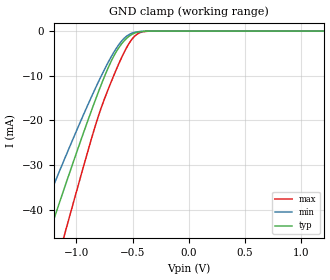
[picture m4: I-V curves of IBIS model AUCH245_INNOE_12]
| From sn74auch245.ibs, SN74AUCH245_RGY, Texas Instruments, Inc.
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[Model]   AUCH245_INNOE_12
Model_type  Input
Vinl=0.385
Vinh=0.845
| variable   typ   min   max
C_comp   2.61pF   2.17pF   3.02pF
[Temperature Range]   40   100   -40
| Ambient temperature   25   85   -40
[Voltage range]   1.2   1.1   1.3
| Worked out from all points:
|   GND clamp passes 1 mA (typ) near -0.52 V on its own axis
[GND Clamp]
| AUCH245_INNOE_12
|   Voltage   I(typ)   I(min)   I(max)
-3.6V     -229.3mA   -192.6mA   -273mA
-1.395V   -56.97mA   -46.56mA   -72.2mA
-1.345V   -53.15mA   -43.42mA   -67.61mA
-1.255V   -46.32mA   -37.82mA   -59.35mA
-1.21V    -42.92mA   -35.05mA   -55.23mA
-1.09V    -33.97mA   -27.77mA   -44.25mA
-835mV    -15.73mA   -13.06mA   -21.55mA
-700mV    -7.296mA   -6.219mA   -11.99mA
-590mV    -2.635mA   -2.022mA   -5.543mA
-465mV    -313.8uA   -199.3uA   -804.4uA
-330mV    -7.615uA   -7.142uA   -10.28uA
1.2V      207.9pA    721.9pA    28.54pA
